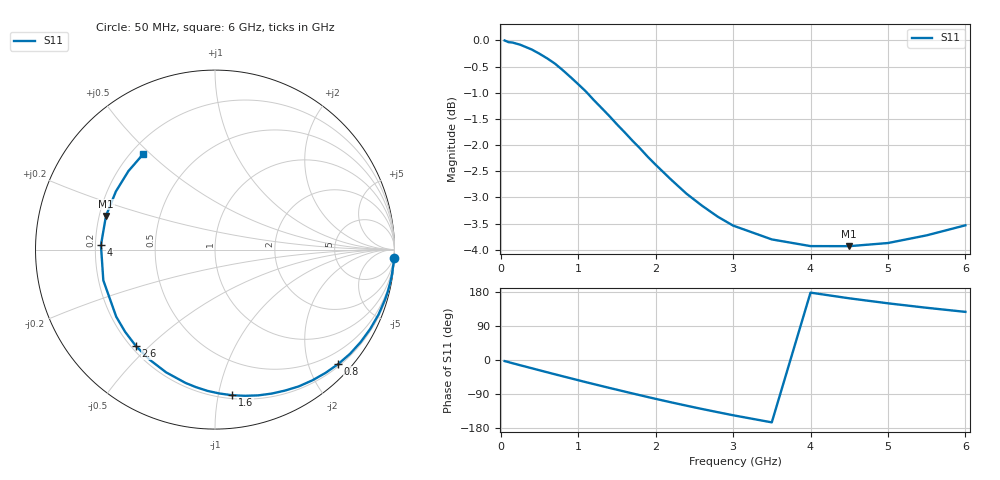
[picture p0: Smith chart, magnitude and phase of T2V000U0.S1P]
! SIEMENS Discrete & RF Semiconductors
! BAS70-04W
! Si Schottky Diode in SOT323
! VR = 0 V
! S-Parameters:  November  1997
# GHz  S  MA  R  50
!  f  S11
! GHz  MAG  ANG
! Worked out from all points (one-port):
!   34 points, 50 MHz to 6 GHz, reference 50 ohm
!   lowest |S11| = -3.9 dB at 4.5 GHz (marker M1), VSWR 4.49, Z = 11.4 + j7.18 ohm
!   |S11| at or under -10 dB: nowhere
!   S11 on the Smith chart (normalised r, x): 50 MHz: 0, -41; 800 MHz: 0.24, -2.53; 1.6 GHz: 0.23, -1.10; 2.6 GHz: 0.22, -0.46; 4 GHz: 0.22, +0.02; 6 GHz: 0.25, +0.47
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0.05  1 -2.8
0.2  0.9931 -11.0
0.3  0.9873 -16.4
0.4  0.9803 -21.7
0.5  0.9712 -27.1
0.6  0.9613 -32.4
0.7  0.9503 -37.7
0.8  0.9368 -42.9
0.9  0.9227 -48.1
1  0.9083 -53.3
1.1  0.8937 -58.5
1.2  0.8773 -63.5
1.3  0.8622 -68.5
1.4  0.8471 -73.5
1.6  0.817 -83.3
1.8  0.7884 -93.0
2  0.7607 -102.5
2.2  0.7361 -111.7
2.4  0.7136 -120.6
2.6  0.695 -129.3
2.8  0.6786 -137.6
3  0.6653 -145.8
3.5  0.6454 -164.6
4  0.6359 177.8
4.5  0.6359 162.8
5  0.6403 149.6
5.5  0.6512 137.8
6  0.6657 127.0
